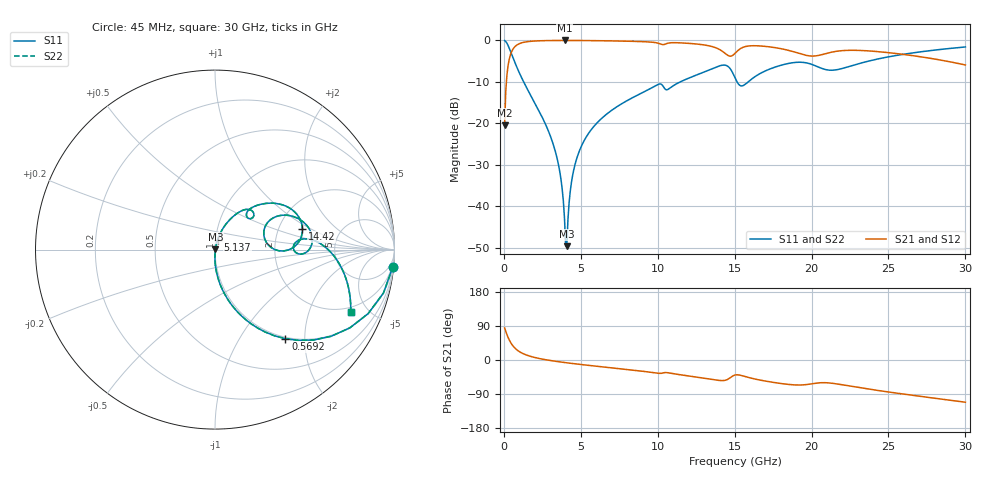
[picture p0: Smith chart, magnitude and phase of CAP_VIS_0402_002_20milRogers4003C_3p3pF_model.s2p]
! S-parameter model data by Modelithics Inc.  support@modelithics.com  813-866-6335  Tampa FL USA
! S-Parameter data specifications:
! Substrate: 20-mil Rogers 4003C, substrate thickness, H=0.508mm, Dielectric constant, Er=3.75
! PCB Mounting Pad Footprint: Pad width, PadW=0.50mm , Pad length, PadL=0.50mm , Pad gap, PadG (edge-to-edge)=0.40mm , Reference planes=1.4mm apart
! Created Wed Nov 18 12:46:41 2015
# hz S ma R 50
! 2 Port Network Data from SP1.SP block
! freq  magS11  angS11  magS21  angS21  magS12  angS12  magS22  angS22
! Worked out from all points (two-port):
!   401 points, 45 MHz to 30 GHz, reference 50 ohm
!   highest |S21| = -0.02 dB at 3.939 GHz (marker M1); lowest = -20.5 dB at 45 MHz (marker M2)
!   |S21| within 3 dB of the highest: 470.2 MHz to 14.34 GHz (13.87 GHz wide, 187 % of centre); 15.05 GHz to 19.09 GHz (4.038 GHz wide, 23.7 % of centre)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
!   lowest |S11| = -49.6 dB at 4.089 GHz (marker M3), VSWR 1.01, Z = 50.3 + j0.186 ohm
!   |S11| at or under -10 dB: 1.283 GHz to 11.46 GHz (10.18 GHz wide, 160 % of centre); 15.16 GHz to 15.88 GHz (724.2 MHz wide, 4.67 % of centre)
!   |S22| runs from -49.6 to 0.0 dB; largest |S21 - S12| = 0
!   S11 on the Smith chart (normalised r, x): 45 MHz: 1, -21; 569.2 MHz: 0.97, -1.61; 5.137 GHz: 1.02, +0.12; 14.42 GHz: 2.72, +0.83; 30 GHz: 1.69, -3.85
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4.5e7  0.9955 -5.5  0.09442 84.5  0.09442 84.5  0.9955 -5.5
2.696625e8  0.8683 -30.2  0.4956 59.8  0.4956 59.8  0.8683 -30.2
5.692125e8  0.6326 -51.7  0.7737 38.2  0.7737 38.2  0.6326 -51.7
1.318088e9  0.3068 -74.2  0.9504 15.5  0.9504 15.5  0.3068 -74.2
3.190275e9  0.0572 -90.2  0.9961 -2.4  0.9961 -2.4  0.0572 -90.2
3.6396e9  0.02571 -89.8  0.9972 -5.0  0.9972 -5.0  0.02571 -89.8
3.93915e9  0.00717 -76.6  0.9974 -6.7  0.9974 -6.7  0.00717 -76.6
4.088925e9  0.003328 33.7  0.9974 -7.4  0.9974 -7.4  0.003328 33.7
4.463362e9  0.02347 74.2  0.997 -9.3  0.997 -9.3  0.02347 74.2
5.062462e9  0.05452 74.8  0.9955 -12.2  0.9955 -12.2  0.05452 74.8
5.13735e9  0.05823 74.7  0.9953 -12.5  0.9953 -12.5  0.05823 74.7
6.784875e9  0.1341 68.6  0.9872 -19.8  0.9872 -19.8  0.1341 68.6
1.007992e10  0.2973 47.8  0.9188 -35.2  0.9188 -35.2  0.2973 47.8
1.330009e10  0.4381 35.5  0.862 -49.6  0.862 -49.6  0.4381 35.5
1.44234e10  0.5007 13.3  0.6872 -53.1  0.6872 -53.1  0.5007 13.3
1.50225e10  0.3545 -1.0  0.6979 -39.7  0.6979 -39.7  0.3545 -1.0
1.554671e10  0.2854 17.8  0.8252 -42.1  0.8252 -42.1  0.2854 17.8
1.711935e10  0.4389 25.9  0.8415 -56.5  0.8415 -56.5  0.4389 25.9
2.003996e10  0.5119 -1.4  0.647 -62.7  0.647 -62.7  0.5119 -1.4
2.16126e10  0.4422 3.8  0.7385 -62.9  0.7385 -62.9  0.4422 3.8
2.505742e10  0.6361 -0.5  0.7093 -84.7  0.7093 -84.7  0.6361 -0.5
3e10  0.8326 -24.8  0.5053 -111.5  0.5053 -111.5  0.8326 -24.8
